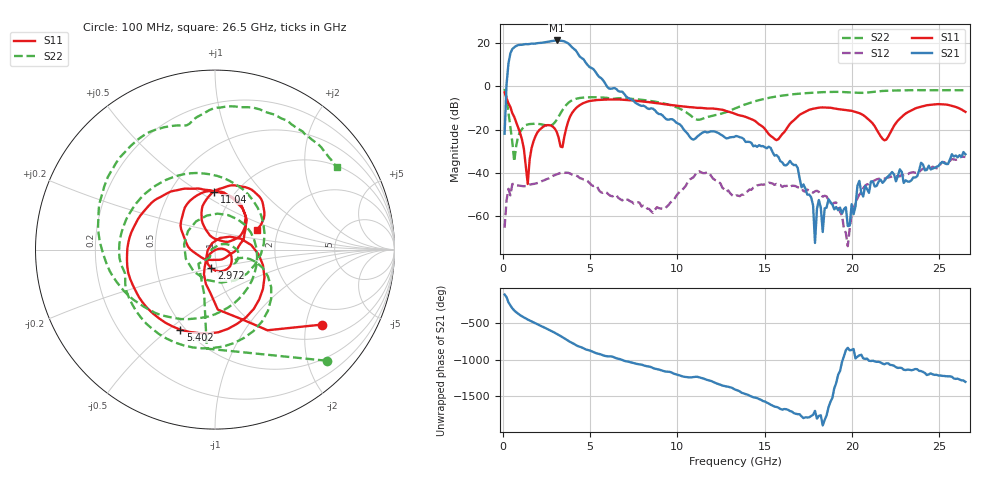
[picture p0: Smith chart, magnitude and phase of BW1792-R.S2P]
!Agilent Technologies,N5242A,MY48420835,A.09.90.17
!Agilent N5242A: A.09.90.17
!Date: Monday, August 22, 2016 16:41:50
!Correction: S11(Full 2 Port(1,2))
!S21(Full 2 Port(1,2))
!S12(Full 2 Port(1,2))
!S22(Full 2 Port(1,2))
!S2P File: Measurements: S11, S21, S12, S22:
# Hz S  dB  R 50
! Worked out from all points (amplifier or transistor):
!   240 points, 100 MHz to 26.5 GHz, reference 50 ohm
!   highest |S21| = 21.2 dB at 3.082 GHz (marker M1)
!   |S21| within 3 dB of that: 678.1 MHz to 3.947 GHz (3.269 GHz wide, 141 % of centre)
!   unconditionally stable (mu >= 1): start of sweep to end of sweep
!   at 4.518 GHz: K = 8.96, MAG = 15.3 dB, |S12| = -42.6 dB
!   at 13.36 GHz: K = 1950.45, MAG = -22.2 dB, |S12| = -50.3 dB
!   at 26.5 GHz: K = 240.16, MAG = -26.2 dB, |S12| = -32.6 dB
!   S11 on the Smith chart (normalised r, x): 100 MHz: 1.39, -2.49; 2.972 GHz: 0.94, -0.20; 5.402 GHz: 0.47, -0.55; 11.04 GHz: 0.81, +0.58; 26.5 GHz: 1.56, +0.37
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1e8  -2.73 -34.9  -21.83 -114.2  -65.24 60.1  -1.13 -44.9
2.104603e8  -5.41 -56.9  0.86 -149.0  -52.63 102.4  -5.14 -94.7
3.209205e8  -7.80 -70.2  10.64 139.6  -47.28 32.9  -11.90 -103.8
5.41841e8  -12.38 -96.4  17.26 57.8  -45.04 32.6  -25.70 -123.6
8.732218e8  -18.93 -120.6  19.09 -14.8  -45.74 -7.3  -23.04 25.8
1.204603e9  -28.82 -139.9  19.44 -64.8  -46.11 -23.3  -18.70 2.1
1.535983e9  -33.59 11.8  19.62 -106.7  -45.33 -34.9  -17.37 -16.1
1.977824e9  -21.23 -13.7  19.99 -157.5  -44.58 -51.5  -17.31 -30.3
2.309205e9  -18.62 -38.5  20.29 165.5  -43.52 -65.1  -17.71 -36.1
2.640586e9  -17.86 -66.1  20.70 127.4  -42.45 -80.4  -18.20 -32.5
2.971967e9  -19.46 -100.9  21.15 86.6  -40.96 -100.9  -16.66 -18.6
3.082427e9  -20.89 -115.9  21.24 72.1  -40.58 -108.4  -15.43 -15.5
3.524268e9  -23.05 67.0  20.81 10.6  -39.80 -143.0  -9.65 -26.7
3.966109e9  -12.24 -6.3  18.07 -51.5  -40.75 -179.6  -6.39 -56.9
4.51841e9  -8.07 -56.8  13.15 -113.1  -42.57 143.4  -5.22 -91.4
5.402092e9  -6.26 -113.4  5.57 164.8  -46.26 95.3  -4.99 -132.9
8.93682e9  -7.80 127.6  -12.75 -53.7  -56.20 14.4  -7.36 98.3
1.103556e10  -9.81 90.5  -24.04 -152.1  -40.60 -65.0  -15.12 -105.9
1.335523e10  -12.88 42.7  -22.88 29.8  -50.34 6.0  -9.93 -71.0
1.777364e10  -10.30 117.3  -54.90 51.0  -49.05 97.2  -2.84 145.8
2.219205e10  -21.45 110.0  -40.58 9.4  -41.81 26.0  -1.92 84.7
2.65e10  -11.75 25.5  -31.31 139.2  -32.61 170.7  -1.73 33.9
